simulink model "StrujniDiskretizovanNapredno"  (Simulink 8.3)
settings: Solver=ode45  StartTime=0.0  StopTime=5  MaxStep=50e-6  RelTol=1e-3
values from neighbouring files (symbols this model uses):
  DELTA = 50    [StrujniDiskretizovanNapredno_parametri.m]
  Ib = 726    [StrujniDiskretizovanNapredno_parametri.m]
  k = 1    [StrujniDiskretizovanNapredno_parametri.m]
  Ki = Kp * K/Tpwm    [StrujniDiskretizovanNapredno_parametri.m]
  Kinv = Vdc/sqrt(3)    [StrujniDiskretizovanNapredno_parametri.m]
  Kp = (1-exp(-lambda*T))/(Kps*(exp(T/Tsigma)-1)*(1+n*(1-exp(-lambda*T))))    [StrujniDiskretizovanNapredno_parametri.m]
  Ks = 1/Rs    (= 222.222222222)    [StrujniDiskretizovanNapredno_parametri.m]
  Lsigma = Tsigma * Rs    (= 5.51900826446e-05)    [StrujniDiskretizovanNapredno_parametri.m]
  T = Tpwm    (= 6.60022440763e-05)    [StrujniDiskretizovanNapredno_parametri.m]
  T0 = 0    [StrujniDiskretizovanNapredno_parametri.m]
  T1 = 10e-3    (= 0.01)    [StrujniDiskretizovanNapredno_parametri.m]
  T2 = 20e-3    (= 0.02)    [StrujniDiskretizovanNapredno_parametri.m]
  T3 = 30e-3    (= 0.03)    [StrujniDiskretizovanNapredno_parametri.m]
  T4 = 40e-3    (= 0.04)    [StrujniDiskretizovanNapredno_parametri.m]
  Tsigma = sigma*Ts    (= 0.0122644628099)    [StrujniDiskretizovanNapredno_parametri.m]
  Vh = inf    [StrujniDiskretizovanNapredno_parametri.m]
  Vl = -inf    [StrujniDiskretizovanNapredno_parametri.m]
  wdq = 0    [StrujniDiskretizovanNapredno_parametri.m]
  wxl = wdq*Lsigma/Kinv*Ib    [StrujniDiskretizovanNapredno_parametri.m]
libraries: simulink x4

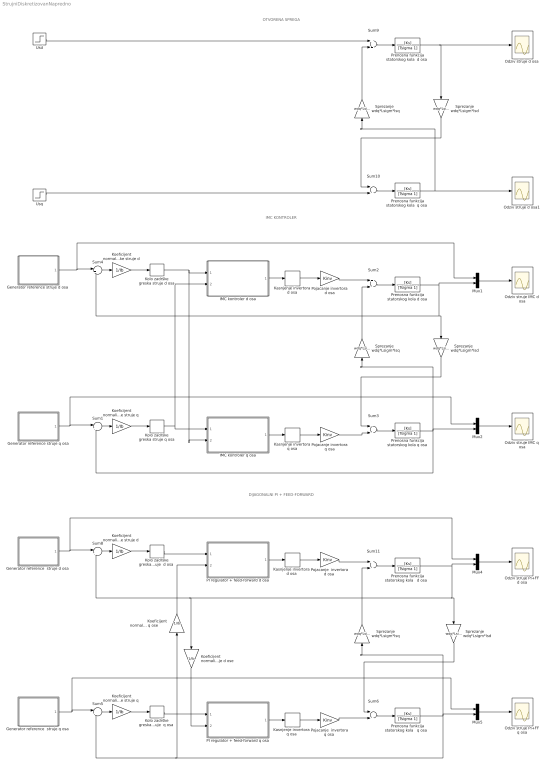
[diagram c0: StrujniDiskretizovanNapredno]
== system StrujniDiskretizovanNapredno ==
  note: IMC KONTROLER
  note: OTVORENA SPREGA
  note: DIJAGONALNI PI + FEED-FORWARD
  "    Sprezanje  wdq*Lsigm*Isd " : Gain  Gain=wdq*Lsigma
  "    Sprezanje      wdq*Lsigm*Isq" : Gain  Gain=wdq*Lsigma
  "   Sprezanje wdq*Lsigm*Isd" : Gain  Gain=wdq*Lsigma
  "   Sprezanje    wdq*Lsigm*Isq" : Gain  Gain=wdq*Lsigma
  "   Sprezanje     wdq*Lsigm*Isq " : Gain  Gain=wdq*Lsigma
  "  Sprezanje    wdq*Lsigm*Isd" : Gain  Gain=wdq*Lsigma
  "Generator reference  struje d osa " : Subsystem
  "Generator reference  struje q osa " : Subsystem
  "Generator reference struje d osa " : Subsystem
  Generator reference struje q osa : Subsystem
  IMC kontroler d osa : Subsystem
  IMC kontroler q osa : Subsystem
  "Kasnjenje invertora  d osa " : Delay  DelayLength=1  SampleTime=T
  "Kasnjenje invertora  q osa " : Delay  DelayLength=1  SampleTime=T
  Kasnjenje invertora d osa : Delay  DelayLength=1  SampleTime=T
  Kasnjenje invertora q osa : Delay  DelayLength=1  SampleTime=T
  "Koeficijent normalizacije         struje d ose   " : Gain  Gain=1/Ib
  "Koeficijent normalizacije   greske struje q " : Gain  Gain=1/Ib
  "Koeficijent normalizacije  greske struje d " : Gain  Gain=1/Ib
  "Koeficijent normalizacije  greske struje q " : Gain  Gain=1/Ib
  Koeficijent normalizacije greske struje d : Gain  Gain=1/Ib
  "Koeficijent normalizacije struje q ose       " : Gain  Gain=1/Ib
  "Kolo zadrške greska struje  d osa " : ZeroOrderHold  SampleTime=T
  "Kolo zadrške greska struje  q osa " : ZeroOrderHold  SampleTime=T
  Kolo zadrške greska struje d osa : ZeroOrderHold  SampleTime=T
  Kolo zadrške greska struje q osa : ZeroOrderHold  SampleTime=T
  Mux{1..2,4..5} (4 alike) : Mux  Inputs=2
  Odziv struje d osa : Scope
  Odziv struje d osa1 : Scope
  Odziv struje IMC d osa : Scope
  Odziv struje IMC q osa : Scope
  Odziv struje PI+FF d osa : Scope
  Odziv struje PI+FF q osa : Scope
  PI regulator + feed-forward d osa : Subsystem
  PI regulator + feed-forward q osa : Subsystem
  "Pojacanje  invertora d osa " : Gain  Gain=Kinv
  "Pojacanje  invertora q osa " : Gain  Gain=Kinv
  Pojacanje invertora d osa : Gain  Gain=Kinv
  Pojacanje invertora q osa : Gain  Gain=Kinv
  "Prenosna funkcija statorskog kola   d osa  " : TransferFcn  Numerator=[Ks]  Denominator=[Tsigma 1]
  "Prenosna funkcija statorskog kola   q osa  " : TransferFcn  Numerator=[Ks]  Denominator=[Tsigma 1]
  "Prenosna funkcija statorskog kola  d osa " : TransferFcn  Numerator=[Ks]  Denominator=[Tsigma 1]
  "Prenosna funkcija statorskog kola  q osa " : TransferFcn  Numerator=[Ks]  Denominator=[Tsigma 1]
  Prenosna funkcija statorskog kola d osa : TransferFcn  Numerator=[Ks]  Denominator=[Tsigma 1]
  Prenosna funkcija statorskog kola q osa : TransferFcn  Numerator=[Ks]  Denominator=[Tsigma 1]
  Sum{1,4..5,8} (4 alike) : Sum  Inputs=|+-
  Sum10 : Sum  Inputs=-+
  Sum11 : Sum
  Sum2 : Sum
  Sum3 : Sum  Inputs=-+
  Sum6 : Sum  Inputs=-+
  Sum9 : Sum
  Usd : Step  Time=1.5  After=0.1  SampleTime=0
  Usq : Step  Time=2.5  After=0.1  SampleTime=0
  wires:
  Mux1/1 -> Odziv struje IMC d osa/1
  Kasnjenje invertora d osa/1 -> Pojacanje invertora d osa/1
  Sum4/1 -> Koeficijent normalizacije greske struje d/1
  Prenosna funkcija statorskog kola d osa/1 -> Sum4/2, "   Sprezanje wdq*Lsigm*Isd"/1, Mux1/2
  "Generator reference struje d osa "/1(Iref) -> Sum4/1, Mux1/1
  Koeficijent normalizacije greske struje d/1 -> Kolo zadrške greska struje d osa/1
  IMC kontroler d osa/1(Vref) -> Kasnjenje invertora d osa/1
  Kolo zadrške greska struje d osa/1 -> IMC kontroler d osa/1(ed), IMC kontroler q osa/2(ed)
  Kasnjenje invertora q osa/1 -> Pojacanje invertora q osa/1
  Sum1/1 -> "Koeficijent normalizacije  greske struje q "/1
  Prenosna funkcija statorskog kola q osa/1 -> "   Sprezanje    wdq*Lsigm*Isq"/1, Sum1/2, Mux2/2
  Generator reference struje q osa/1(Iref) -> Mux2/1, Sum1/1
  "Koeficijent normalizacije  greske struje q "/1 -> Kolo zadrške greska struje q osa/1
  IMC kontroler q osa/1(Vref) -> Kasnjenje invertora q osa/1
  Kolo zadrške greska struje q osa/1 -> IMC kontroler q osa/1(eq), IMC kontroler d osa/2(eq)
  Pojacanje invertora d osa/1 -> Sum2/1
  "   Sprezanje    wdq*Lsigm*Isq"/1 -> Sum2/2
  Mux4/1 -> Odziv struje PI+FF d osa/1
  "Kasnjenje invertora  d osa "/1 -> "Pojacanje  invertora d osa "/1
  Sum8/1 -> "Koeficijent normalizacije  greske struje d "/1
  "Generator reference  struje d osa "/1(Iref) -> Mux4/1, Sum8/1
  "Koeficijent normalizacije  greske struje d "/1 -> "Kolo zadrške greska struje  d osa "/1
  "Kolo zadrške greska struje  d osa "/1 -> PI regulator + feed-forward d osa/1(ed)
  Mux5/1 -> Odziv struje PI+FF q osa/1
  "Kasnjenje invertora  q osa "/1 -> "Pojacanje  invertora q osa "/1
  Sum5/1 -> "Koeficijent normalizacije   greske struje q "/1
  "Generator reference  struje q osa "/1(Iref) -> Sum5/1, Mux5/1
  "Koeficijent normalizacije   greske struje q "/1 -> "Kolo zadrške greska struje  q osa "/1
  "Kolo zadrške greska struje  q osa "/1 -> PI regulator + feed-forward q osa/1(eq)
  "Pojacanje  invertora d osa "/1 -> Sum11/1
  "    Sprezanje      wdq*Lsigm*Isq"/1 -> Sum11/2
  "Pojacanje  invertora q osa "/1 -> Sum6/2
  "Prenosna funkcija statorskog kola   q osa  "/1 -> Sum5/2, "Koeficijent normalizacije struje q ose       "/1, Mux5/2, "    Sprezanje      wdq*Lsigm*Isq"/1
  "Koeficijent normalizacije struje q ose       "/1 -> PI regulator + feed-forward d osa/2(eq)
  "Koeficijent normalizacije         struje d ose   "/1 -> PI regulator + feed-forward q osa/2(ed)
  Mux2/1 -> Odziv struje IMC q osa/1
  PI regulator + feed-forward d osa/1(Vref) -> "Kasnjenje invertora  d osa "/1
  PI regulator + feed-forward q osa/1(Vref) -> "Kasnjenje invertora  q osa "/1
  Sum3/1 -> Prenosna funkcija statorskog kola q osa/1
  Pojacanje invertora q osa/1 -> Sum3/2
  Sum2/1 -> Prenosna funkcija statorskog kola d osa/1
  "   Sprezanje wdq*Lsigm*Isd"/1 -> Sum3/1
  "Prenosna funkcija statorskog kola  d osa "/1 -> Odziv struje d osa/1, "    Sprezanje  wdq*Lsigm*Isd "/1
  "Prenosna funkcija statorskog kola  q osa "/1 -> "   Sprezanje     wdq*Lsigm*Isq "/1, Odziv struje d osa1/1
  Usd/1 -> Sum9/1
  "   Sprezanje     wdq*Lsigm*Isq "/1 -> Sum9/2
  Sum10/1 -> "Prenosna funkcija statorskog kola  q osa "/1
  Usq/1 -> Sum10/2
  Sum9/1 -> "Prenosna funkcija statorskog kola  d osa "/1
  "    Sprezanje  wdq*Lsigm*Isd "/1 -> Sum10/1
  Sum11/1 -> "Prenosna funkcija statorskog kola   d osa  "/1
  "Prenosna funkcija statorskog kola   d osa  "/1 -> Sum8/2, "Koeficijent normalizacije         struje d ose   "/1, "  Sprezanje    wdq*Lsigm*Isd"/1, Mux4/2
  "  Sprezanje    wdq*Lsigm*Isd"/1 -> Sum6/1
  Sum6/1 -> "Prenosna funkcija statorskog kola   q osa  "/1

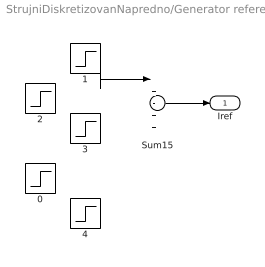
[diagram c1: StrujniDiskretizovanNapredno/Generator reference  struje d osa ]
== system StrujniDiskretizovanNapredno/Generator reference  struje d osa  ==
  0 : Step  Time=T0  After=DELTA  SampleTime=0
  1 : Step  Time=1.5  After=DELTA/3  SampleTime=0
  2 : Step  Time=T2  After=DELTA  SampleTime=0
  3 : Step  Time=T3  After=DELTA  SampleTime=0
  4 : Step  Time=T4  After=DELTA  SampleTime=0
  Sum15 : Sum  Inputs=|+-++-
  Iref : Outport
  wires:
  Sum15/1 -> Iref/1
  1/1 -> Sum15/1

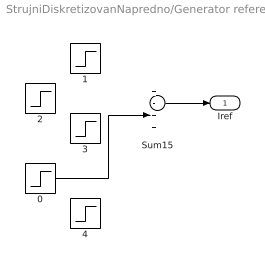
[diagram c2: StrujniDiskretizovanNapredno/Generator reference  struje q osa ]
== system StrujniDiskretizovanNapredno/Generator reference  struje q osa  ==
  0 : Step  Time=2.5  After=DELTA  SampleTime=0
  1 : Step  Time=T1  After=DELTA  SampleTime=0
  2 : Step  Time=T2  After=DELTA  SampleTime=0
  3 : Step  Time=T3  After=DELTA  SampleTime=0
  4 : Step  Time=T4  After=DELTA  SampleTime=0
  Sum15 : Sum  Inputs=|+-++-
  Iref : Outport
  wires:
  0/1 -> Sum15/4
  Sum15/1 -> Iref/1

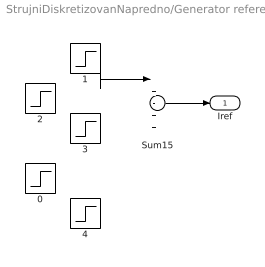
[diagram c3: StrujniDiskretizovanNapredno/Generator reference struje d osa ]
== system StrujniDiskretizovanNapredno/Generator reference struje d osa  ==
  0 : Step  Time=T0  After=DELTA  SampleTime=0
  1 : Step  Time=1.5  After=DELTA/3  SampleTime=0
  2 : Step  Time=T2  After=DELTA  SampleTime=0
  3 : Step  Time=T3  After=DELTA  SampleTime=0
  4 : Step  Time=T4  After=DELTA  SampleTime=0
  Sum15 : Sum  Inputs=|+-++-
  Iref : Outport
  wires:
  1/1 -> Sum15/1
  Sum15/1 -> Iref/1

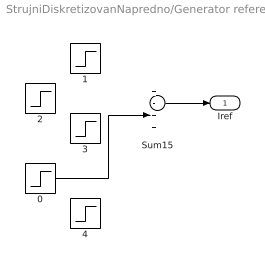
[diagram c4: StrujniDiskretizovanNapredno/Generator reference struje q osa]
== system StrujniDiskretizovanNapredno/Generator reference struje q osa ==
  0 : Step  Time=2.5  After=DELTA  SampleTime=0
  1 : Step  Time=T1  After=DELTA  SampleTime=0
  2 : Step  Time=T2  After=DELTA  SampleTime=0
  3 : Step  Time=T3  After=DELTA  SampleTime=0
  4 : Step  Time=T4  After=DELTA  SampleTime=0
  Sum15 : Sum  Inputs=|+-++-
  Iref : Outport
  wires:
  Sum15/1 -> Iref/1
  0/1 -> Sum15/4

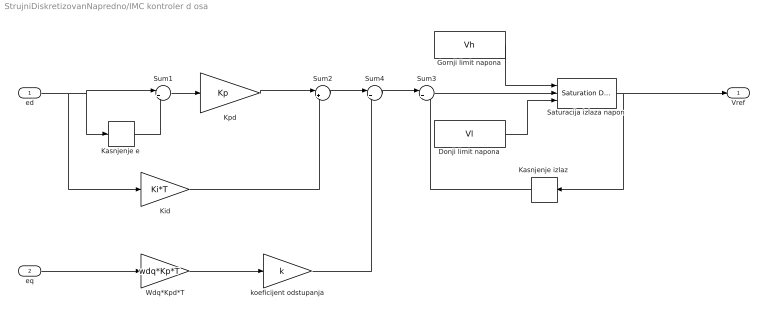
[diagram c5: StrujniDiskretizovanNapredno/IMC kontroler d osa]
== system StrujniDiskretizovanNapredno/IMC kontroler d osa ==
  ed : Inport
  eq : Inport  Port=2
  Donji limit napona : Constant  Value=Vl  SampleTime=T
  Gornji limit napona : Constant  Value=Vh  SampleTime=T
  Kasnjenje izlaz : Delay  DelayLength=1  SampleTime=T
  Kasnjenje e : Delay  DelayLength=1  SampleTime=T
  Kid : Gain  Gain=Ki*T  SampleTime=T
  Kpd : Gain  Gain=Kp  SampleTime=T
  Saturacija izlaza napon : simulink/Discontinuities/Saturation Dynamic  OutMin=[]  OutMax=[]  OutDataTypeStr=Inherit: Same as second input  OutDataType=fixdt(1, 16)  OutScaling=2^-10  DoSatur=off
  Sum1 : Sum  Inputs=|+-  SampleTime=T
  Sum2 : Sum  Inputs=|++  SampleTime=T
  Sum3 : Sum  Inputs=|++  SampleTime=T
  Sum4 : Sum  Inputs=|+-  SampleTime=T
  Wdq*Kpd*T : Gain  Gain=wdq*Kp*T  SampleTime=T
  koeficijent odstupanja : Gain  Gain=k  SampleTime=T
  Vref : Outport
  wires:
  Gornji limit napona/1 -> Saturacija izlaza napon/1
  ed/1 -> Sum1/1, Kasnjenje e/1, Kid/1
  Donji limit napona/1 -> Saturacija izlaza napon/3
  Sum1/1 -> Kpd/1
  Kid/1 -> Sum2/2
  Kpd/1 -> Sum2/1
  Sum3/1 -> Saturacija izlaza napon/2
  Kasnjenje izlaz/1 -> Sum3/2
  Saturacija izlaza napon/1 -> Vref/1, Kasnjenje izlaz/1
  Kasnjenje e/1 -> Sum1/2
  Sum2/1 -> Sum4/1
  Sum4/1 -> Sum3/1
  eq/1 -> Wdq*Kpd*T/1
  Wdq*Kpd*T/1 -> koeficijent odstupanja/1
  koeficijent odstupanja/1 -> Sum4/2

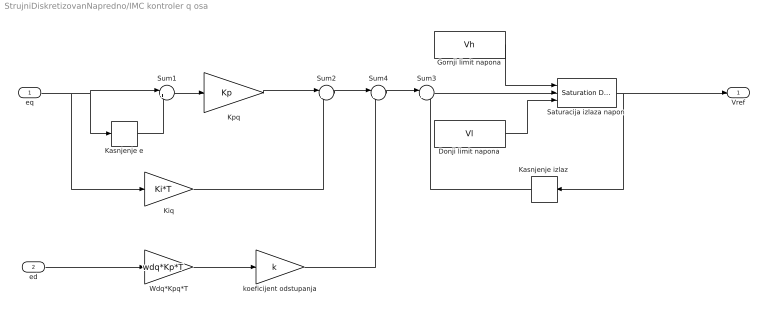
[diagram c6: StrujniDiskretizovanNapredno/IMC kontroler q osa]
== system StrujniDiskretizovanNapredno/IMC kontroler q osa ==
  eq : Inport
  ed : Inport  Port=2
  Donji limit napona : Constant  Value=Vl  SampleTime=T
  Gornji limit napona : Constant  Value=Vh  SampleTime=T
  Kasnjenje izlaz : Delay  DelayLength=1  SampleTime=T
  Kasnjenje e : Delay  DelayLength=1  SampleTime=T
  Kiq : Gain  Gain=Ki*T  SampleTime=T
  Kpq : Gain  Gain=Kp  SampleTime=T
  Saturacija izlaza napon : simulink/Discontinuities/Saturation Dynamic  OutMin=[]  OutMax=[]  OutDataTypeStr=Inherit: Same as second input  OutDataType=fixdt(1, 16)  OutScaling=2^-10  DoSatur=off
  Sum1 : Sum  Inputs=|+-  SampleTime=T
  Sum2 : Sum  Inputs=|++  SampleTime=T
  Sum3 : Sum  Inputs=|++  SampleTime=T
  Sum4 : Sum  Inputs=|++  SampleTime=T
  Wdq*Kpq*T : Gain  Gain=wdq*Kp*T  SampleTime=T
  koeficijent odstupanja : Gain  Gain=k  SampleTime=T
  Vref : Outport
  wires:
  Kasnjenje e/1 -> Sum1/2
  Saturacija izlaza napon/1 -> Kasnjenje izlaz/1, Vref/1
  Kasnjenje izlaz/1 -> Sum3/2
  Sum3/1 -> Saturacija izlaza napon/2
  Kpq/1 -> Sum2/1
  Kiq/1 -> Sum2/2
  Sum1/1 -> Kpq/1
  Donji limit napona/1 -> Saturacija izlaza napon/3
  eq/1 -> Kiq/1, Kasnjenje e/1, Sum1/1
  Gornji limit napona/1 -> Saturacija izlaza napon/1
  ed/1 -> Wdq*Kpq*T/1
  Sum2/1 -> Sum4/1
  Sum4/1 -> Sum3/1
  Wdq*Kpq*T/1 -> koeficijent odstupanja/1
  koeficijent odstupanja/1 -> Sum4/2

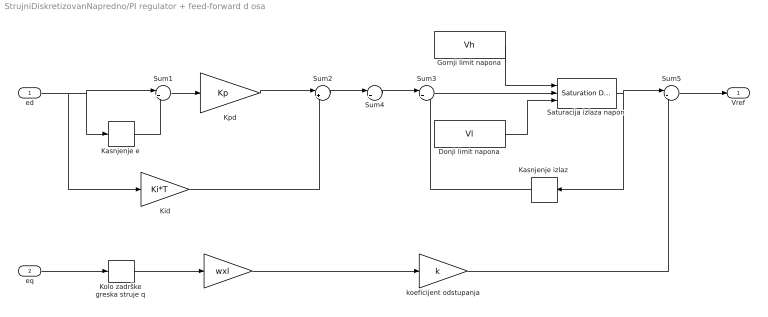
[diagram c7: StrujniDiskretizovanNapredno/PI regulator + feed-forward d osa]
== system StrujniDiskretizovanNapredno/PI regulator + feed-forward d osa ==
  ed : Inport
  eq : Inport  Port=2
  "  " : Gain  Gain=wxl  SampleTime=T
  Donji limit napona : Constant  Value=Vl  SampleTime=T
  Gornji limit napona : Constant  Value=Vh  SampleTime=T
  Kasnjenje izlaz : Delay  DelayLength=1  SampleTime=T
  Kasnjenje e : Delay  DelayLength=1  SampleTime=T
  Kid : Gain  Gain=Ki*T  SampleTime=T
  Kolo zadrške greska struje q : ZeroOrderHold  SampleTime=T
  Kpd : Gain  Gain=Kp  SampleTime=T
  Saturacija izlaza napon : simulink/Discontinuities/Saturation Dynamic  OutMin=[]  OutMax=[]  OutDataTypeStr=Inherit: Same as second input  OutDataType=fixdt(1, 16)  OutScaling=2^-10  DoSatur=off
  Sum1 : Sum  Inputs=|+-  SampleTime=T
  Sum2 : Sum  Inputs=|++  SampleTime=T
  Sum3 : Sum  Inputs=|++  SampleTime=T
  Sum4 : Sum  Inputs=|+-  SampleTime=T
  Sum5 : Sum  Inputs=|+-  SampleTime=T
  koeficijent odstupanja : Gain  Gain=k  SampleTime=T
  Vref : Outport
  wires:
  eq/1 -> Kolo zadrške greska struje q/1
  Sum4/1 -> Sum3/1
  Sum2/1 -> Sum4/1
  Kasnjenje e/1 -> Sum1/2
  Saturacija izlaza napon/1 -> Sum5/1, Kasnjenje izlaz/1
  Kasnjenje izlaz/1 -> Sum3/2
  Sum3/1 -> Saturacija izlaza napon/2
  Kpd/1 -> Sum2/1
  Kid/1 -> Sum2/2
  Sum1/1 -> Kpd/1
  Donji limit napona/1 -> Saturacija izlaza napon/3
  ed/1 -> Kid/1, Kasnjenje e/1, Sum1/1
  Gornji limit napona/1 -> Saturacija izlaza napon/1
  Kolo zadrške greska struje q/1 -> "  "/1
  Sum5/1 -> Vref/1
  "  "/1 -> koeficijent odstupanja/1
  koeficijent odstupanja/1 -> Sum5/2

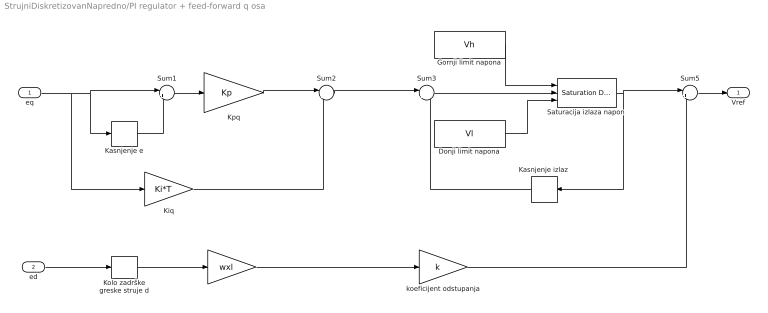
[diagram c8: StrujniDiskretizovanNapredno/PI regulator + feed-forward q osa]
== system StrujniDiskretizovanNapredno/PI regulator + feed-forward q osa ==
  eq : Inport
  ed : Inport  Port=2
  "   " : Gain  Gain=wxl  SampleTime=T
  Donji limit napona : Constant  Value=Vl  SampleTime=T
  Gornji limit napona : Constant  Value=Vh  SampleTime=T
  Kasnjenje izlaz : Delay  DelayLength=1  SampleTime=T
  Kasnjenje e : Delay  DelayLength=1  SampleTime=T
  Kiq : Gain  Gain=Ki*T  SampleTime=T
  Kolo zadrške greske struje d : ZeroOrderHold  SampleTime=T
  Kpq : Gain  Gain=Kp  SampleTime=T
  Saturacija izlaza napon : simulink/Discontinuities/Saturation Dynamic  OutMin=[]  OutMax=[]  OutDataTypeStr=Inherit: Same as second input  OutDataType=fixdt(1, 16)  OutScaling=2^-10  DoSatur=off
  Sum1 : Sum  Inputs=|+-  SampleTime=T
  Sum2 : Sum  Inputs=|++  SampleTime=T
  Sum3 : Sum  Inputs=|++  SampleTime=T
  Sum5 : Sum  Inputs=|++  SampleTime=T
  koeficijent odstupanja : Gain  Gain=k  SampleTime=T
  Vref : Outport
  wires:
  Sum2/1 -> Sum3/1
  ed/1 -> Kolo zadrške greske struje d/1
  Gornji limit napona/1 -> Saturacija izlaza napon/1
  eq/1 -> Sum1/1, Kasnjenje e/1, Kiq/1
  Donji limit napona/1 -> Saturacija izlaza napon/3
  Sum1/1 -> Kpq/1
  Kiq/1 -> Sum2/2
  Kpq/1 -> Sum2/1
  Sum3/1 -> Saturacija izlaza napon/2
  Kasnjenje izlaz/1 -> Sum3/2
  Saturacija izlaza napon/1 -> Sum5/1, Kasnjenje izlaz/1
  Kasnjenje e/1 -> Sum1/2
  Kolo zadrške greske struje d/1 -> "   "/1
  Sum5/1 -> Vref/1
  "   "/1 -> koeficijent odstupanja/1
  koeficijent odstupanja/1 -> Sum5/2
